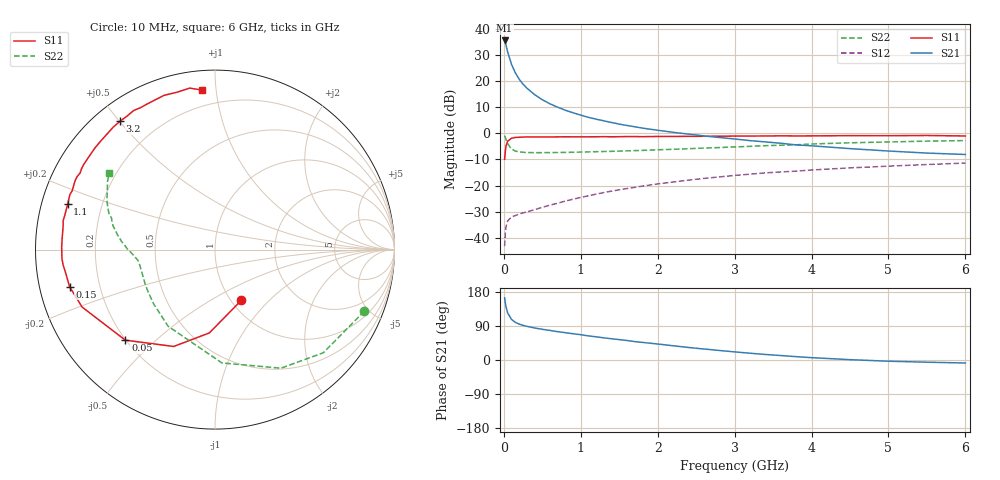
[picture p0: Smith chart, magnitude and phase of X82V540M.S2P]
! SIEMENS Small Signal Semiconductors
! BFP136W
! Si NPN RF Bipolar Junction Transistor in SOT343
! VCE = 2.5 V  IC = 40 mA
! Common Emitter S-Parameters:  September  1994
# GHz  S  MA  R  50
!  f  S11  S21  S12  S22
! GHz  MAG  ANG  MAG  ANG  MAG  ANG  MAG  ANG
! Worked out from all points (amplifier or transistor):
!   40 points, 10 MHz to 6 GHz, reference 50 ohm
!   highest |S21| = 35.6 dB at 10 MHz (marker M1)
!   |S21| within 3 dB of that: start of sweep to 38.29 MHz
!   unconditionally stable (mu >= 1): 663 MHz to 2.86 GHz
!   at 200 MHz: K = 0.50, MSG = 25.8 dB, |S12| = -30.9 dB
!   at 1.5 GHz: K = 1.13, MAG = 10.4 dB, |S12| = -21.6 dB
!   at 6 GHz: K = 0.97, MSG = 1.6 dB, |S12| = -11.4 dB
!   S11 on the Smith chart (normalised r, x): 10 MHz: 1.11, -0.70; 50 MHz: 0.20, -0.40; 150 MHz: 0.09, -0.12; 1.1 GHz: 0.08, +0.15; 3.2 GHz: 0.07, +0.50; 6 GHz: 0.11, +0.92
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0.01  0.318 -62.4  60.24 164.1  0.0069 72.6  0.9002 -22.4
0.02  0.4655 -93.9  54.12 149.9  0.0126 62.3  0.8335 -43.6
0.03  0.5867 -113.1  47.92 138.9  0.0166 53.7  0.7561 -60.9
0.05  0.71 -134.7  36.17 123.9  0.0211 40.4  0.6327 -86.5
0.1  0.8066 -156.6  20.91 107.0  0.025 31.6  0.5006 -121.4
0.15  0.8363 -165.7  14.39 99.3  0.0267 30.5  0.4569 -138.1
0.2  0.8412 -170.6  10.85 94.7  0.0285 31.2  0.4412 -147.6
0.25  0.85 -174.1  8.768 91.4  0.03 33.2  0.4342 -153.6
0.3  0.8541 -176.5  7.332 88.9  0.0312 35.6  0.4292 -157.7
0.4  0.8543 179.2  5.529 84.5  0.0346 39.4  0.4269 -162.9
0.5  0.854 176.0  4.41 81.0  0.0383 43.5  0.4271 -166.3
0.6  0.8541 173.7  3.677 78.0  0.0421 46.5  0.428 -168.4
0.7  0.8565 171.0  3.172 74.7  0.0459 49.2  0.43 -169.8
0.9  0.8583 167.2  2.479 69.2  0.0548 52.3  0.4343 -172.3
1.1  0.8588 162.9  2.025 63.5  0.0637 54.6  0.4416 -173.7
1.5  0.8636 156.0  1.502 53.8  0.0828 56.3  0.4569 -176.3
1.8  0.8641 150.4  1.263 46.5  0.0975 55.6  0.4717 -178.5
2.2  0.8725 143.7  1.048 37.6  0.1169 53.9  0.4946 178.6
3.2  0.8896 126.5  0.726 17.9  0.1652 46.3  0.5637 169.2
4.5  0.9051 108.3  0.51 0.9  0.2181 34.5  0.6601 155.8
5.5  0.9107 98.9  0.419 -5.8  0.2529 26.5  0.71 147.5
6  0.8916 94.6  0.394 -7.9  0.2698 22.1  0.7276 144.0
